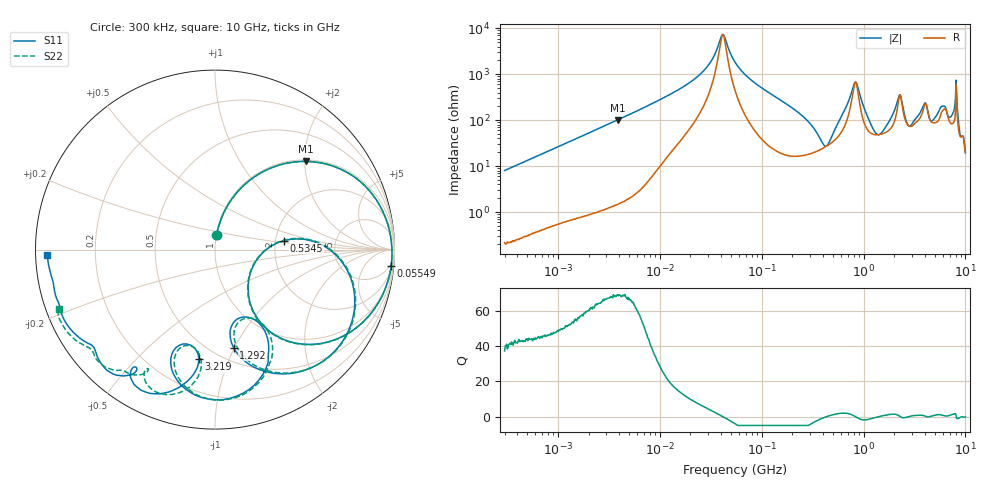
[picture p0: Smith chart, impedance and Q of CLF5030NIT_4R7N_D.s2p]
! S-Parameter Data Generated by TDK Corporation
! Copyright(C) 2019 TDK Corporation.
! All Rights Reserved.
! TDK P/N: CLF5030NIT-4R7N-D (Inductor)
! Property: L=4.7uH at 100kHz
! Size(LxWxT): 5.3x5x2.7mm
! Model Type: s2p (Touchstone File Format Version 1.0)
! Frequency: DC=Yes Start=0.3MHz Stop=10000MHz 802points Log-sweep
! Model Generated on May 10, 2019
! Port Assignments:
!  1 ---@@@--- 2
! Applicable Conditions:
!  Temperature = 25 degC
!  DC Bias Current = 0 A
!  Small Signal Operation
! Terms and conditions regarding TDK Simulation Models
! (1)This simulation model is being provided solely for informational purposes. Please refer to the specifications of the products in terms of detailed characteristics of such products.
! (2)In no event shall TDK Corporation of any of its subsidiaries be liable for any loss or damage arising, directly or indirectly,
!  From any information contained in this simulation model, including, but not limited to loss or damages arising from any inaccuracies, omissions or errors in connection with such information.
! (3)Any and all copyrights on this simulation model are owned by TDK Corporation.
!  Duplication or redistribution of this simulation model without prior written permission from TDK Corporation is prohibited.
! (4)This simulation model is subject to any modification or change without any prior notice.
! (5)Neither TDK Corporation nor any of its subsidiaries shall make any warranty, express or implied,
!  Including but not limited to the correctness, implied warranties of merchantability and fitness for a particular purpose with respect to this simulation models.
! (6)The use of this simulation model shall be deemed to have consented to the terms and conditions hereof.
# Hz S MA R 50
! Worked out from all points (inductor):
!   801 points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, 300 kHz to 10 GHz, reference 50 ohm
!   read as one part in series: L = 4.24 uH near 318.3 kHz
!   highest Q = 68.9 at 3.867 MHz (marker M1), where L = 4.18 uH
!   self-resonance near 41.38 MHz
!   S11 on the Smith chart (normalised r, x): 300 kHz: 1.00, +0.16; 55.49 MHz: 3, -21; 534.5 MHz: 2.23, +0.26; 1.292 GHz: 0.63, -0.99; 3.219 GHz: 0.40, -0.78; 10 GHz: 0.03, -0.02
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300000  0.07997 84.0  0.9945 -4.6  0.9944 -4.6  0.08001 84.1
1713600  0.4066 65.0  0.9065 -24.0  0.9065 -24.0  0.4067 65.0
3866967  0.7068 44.0  0.697 -45.1  0.6972 -45.1  0.7069 44.0
9671944  0.927 19.8  0.3456 -68.3  0.3456 -68.3  0.9271 19.8
2.567637e7  0.9814 4.2  0.09206 -76.9  0.09207 -76.9  0.9814 4.2
4.138262e7  0.9865 -1.6  0.01339 -5.8  0.01338 -5.8  0.9867 -1.6
5.477226e7  0.9856 -5.2  0.05349 70.8  0.0535 70.8  0.9857 -5.2
5.548994e7  0.9854 -5.4  0.05595 71.2  0.05597 71.2  0.9856 -5.4
1.563148e8  0.9185 -25.9  0.337 60.0  0.337 60.0  0.9185 -26.1
3.126428e8  0.5939 -54.4  0.6833 22.6  0.6832 22.6  0.593 -54.7
4.448526e8  0.2344 -31.6  0.7717 -13.9  0.7717 -13.9  0.232 -31.5
5.344909e8  0.3878 7.4  0.6834 -37.6  0.6834 -37.6  0.3881 7.8
8.414386e8  0.8749 -35.0  0.118 -25.5  0.118 -25.5  0.8778 -34.6
1.292013e9  0.5557 -79.3  0.5534 -23.9  0.5535 -23.9  0.5566 -77.3
1.767019e9  0.4673 -59.5  0.5151 -78.2  0.5153 -78.2  0.4906 -57.4
2.294622e9  0.8371 -86.7  0.1269 -78.9  0.1271 -79.1  0.8394 -87.4
3.219363e9  0.6175 -98.4  0.2789 -97.4  0.2778 -97.0  0.5563 -102.7
4.049484e9  0.8829 -116.1  0.1154 -111.8  0.1158 -111.6  0.8521 -108.5
4.807583e9  0.7911 -123.5  0.2076 -123.3  0.2083 -123.4  0.7633 -119.1
6.979804e9  0.8795 -143.6  0.0812 -158.5  0.08096 -158.4  0.8938 -142.7
8.09931e9  0.9204 -160.2  0.00505 -172.3  0.005393 -169.5  0.9467 -153.9
1e10  0.9348 -178.0  0.0328 -84.9  0.03254 -85.5  0.9302 -159.1
